|Texas Instruments Incorporated
| 3-Line To 8-Line decoder/Demultiplexer
| Marketing part#   Digital Voltage Range   Package-type   #pins
| SN74LVC138AD   1.65V - 3.6V   SOIC   16
| SN74LVC138ADBR   1.65V - 3.6V   SSOP   16
| SN74LVC138ADBRE4   1.65V - 3.6V   SSOP   16
| SN74LVC138ADBRG4   1.65V - 3.6V   SSOP   16
| SN74LVC138ADE4   1.65V - 3.6V   SOIC   16
| SN74LVC138ADG4   1.65V - 3.6V   SOIC   16
| SN74LVC138ADGVR   1.65V - 3.6V   TVSOP   16
| SN74LVC138ADGVRE4  1.65V - 3.6V   TVSOP   16
| SN74LVC138ADGVRG4  1.65V - 3.6V   TVSOP   16
| SN74LVC138ADR   1.65V - 3.6V   SOIC   16
| SN74LVC138ADRE4   1.65V - 3.6V   SOIC   16
| SN74LVC138ADRG4   1.65V - 3.6V   SOIC   16
| SN74LVC138ADT   1.65V - 3.6V   SOIC   16
| SN74LVC138ADTE4   1.65V - 3.6V   SOIC   16
| SN74LVC138ADTG4   1.65V - 3.6V   SOIC   16
| SN74LVC138AGQNR   1.65V - 3.6V   BGA MICROSTAR JUNIOR  20
| SN74LVC138ANSR   1.65V - 3.6V   SO   16
| SN74LVC138ANSRE4   1.65V - 3.6V   SO   16
| SN74LVC138ANSRG4   1.65V - 3.6V   SO   16
| SN74LVC138APW   1.65V - 3.6V   TSSOP   16
| SN74LVC138APWE4   1.65V - 3.6V   TSSOP   16
| SN74LVC138APWG4   1.65V - 3.6V   TSSOP   16
| SN74LVC138APWR   1.65V - 3.6V   TSSOP   16
| SN74LVC138APWRE4   1.65V - 3.6V   TSSOP   16
| SN74LVC138APWRG4   1.65V - 3.6V   TSSOP   16
| SN74LVC138APWT   1.65V - 3.6V   TSSOP   16
| SN74LVC138APWTE4   1.65V - 3.6V   TSSOP   16
| SN74LVC138APWTG4   1.65V - 3.6V   TSSOP   16
| SN74LVC138ARGYR   1.65V - 3.6V   VQFN   16
| SN74LVC138ARGYRG4  1.65V - 3.6V   VQFN   16
| SN74LVC138AZQNR   1.65V - 3.6V   BGA MICROSTAR JUNIOR  20
[IBIS Ver]   3.2
[File name]   sn74lvc138a.ibs
[File Rev]   1.0
[Date]   6/21/2012
[Source]
| Texas Instruments Incorporated.
| Analog-eLab Design Center, HPA
| 12500 TI Blvd
| Dallas, TX -75243
| e-mail: elab_scm_ibis@list.ti.com
[Notes]   Revision History:
| Rev 1.0: 6/21/2012
| - Initial version of the model
| - Model generated from simulations in TISPICE
| - Model matched to SPICE simulation
| - C_comp although listed in numerical order of value are
|   obtained from varying PVT conditions. For PVT conditions for
|   each specific value refer the buffer description under
|   respective [Model]. IBIS model user is responsible for using
|   appropriate C_comp to simulate for Signal Integrity.
| - Model names with a trailing _1p8 contains the model for
|   1.8V [1.71V and 1.89V]. Model names with a trailing _3p3
|   contains the model for 3.3V [3.0V and 3.6V].
[Disclaimer]
| This model is designed as an aid for customers of Texas Instruments.
| TI and its licensors and suppliers make no warranties, either expressed
| or implied, with respect to this  model, including the warranties of
| merchantability or fitness for a particular purpose. The model is
| provided solely on an "as is" basis. The entire risk as to its quality
| and performance is with the customer.
[Copyright]
(C) Copyright 2012 Texas Instruments Incorporated.All rights reserved.
|   SN74LVC138ARGY
[Component]   SN74LVC138ARGY
[Manufacturer]   TI
[Package]   |16 VQFN   -  RGY package
|   typ   min   max
R_pkg   0.07181   0.06369   0.08091
L_pkg   1.28975nH   1.12199nH   1.48239nH
C_pkg   0.23145pF   0.21992pF   0.24704pF
[Pin]  signal_name   model_name   R_pin   L_pin   C_pin
1   A   INPUT   0.08031   1.46839nH  0.22398pF
2   B   INPUT   0.08091   1.48239nH  0.23668pF
3   C   INPUT   0.07045   1.26496nH  0.23607pF
4   _G2A   INPUT   0.06569   1.16779nH  0.22308pF
5   _G2B   INPUT   0.06369   1.12697nH  0.22065pF
6   G1   INPUT   0.06587   1.17112nH  0.23290pF
7   Y7   OUTPUT   0.07968   1.45609nH  0.24704pF
8   GND   GND   0.08286   1.52103nH  0.24643pF
9   Y6   OUTPUT   0.07976   1.45197nH  0.23427pF
10   Y5   OUTPUT   0.07984   1.45159nH  0.23652pF
11   Y4   OUTPUT   0.06755   1.19686nH  0.23355pF
12   Y3   OUTPUT   0.06389   1.12199nH  0.22012pF
13   Y2   OUTPUT   0.06405   1.12517nH  0.21992pF
14   Y1   OUTPUT   0.06746   1.19483nH  0.23367pF
15   Y0   OUTPUT   0.07624   1.37643nH  0.24190pF
16   VCC   POWER   0.07919   1.44018nH  0.23234pF
|   SN74LVC138AD
[Component]   SN74LVC138AD
[Manufacturer]   TI
[Package]   |16 SOIC   -  D   package
|   typ   min   max
R_pkg   0.10679   0.08959   0.12155
L_pkg   2.86135nH   2.04402nH   4.29838nH
C_pkg   0.80708pF   0.61580pF   1.19610pF
[Pin]  signal_name   model_name   R_pin   L_pin   C_pin
1   A   INPUT   0.10965   4.21181nH  1.19116pF
2   B   INPUT   0.11559   3.48714nH  0.97723pF
3   C   INPUT   0.10942   2.29983nH  0.63814pF
4   _G2A   INPUT   0.09310   2.09121nH  0.61836pF
5   _G2B   INPUT   0.08959   2.04402nH  0.61580pF
6   G1   INPUT   0.10155   2.19279nH  0.63325pF
7   Y7   OUTPUT   0.11898   3.56208nH  0.96757pF
8   GND   GND   0.11687   4.32168nH  1.19555pF
9   Y6   OUTPUT   0.11525   4.29838nH  1.19610pF
10   Y5   OUTPUT   0.12155   3.59908nH  0.97047pF
11   Y4   OUTPUT   0.10999   2.31319nH  0.63900pF
12   Y3   OUTPUT   0.09528   2.12402nH  0.61985pF
13   Y2   OUTPUT   0.09454   2.11191nH  0.61892pF
14   Y1   OUTPUT   0.10669   2.26123nH  0.63716pF
15   Y0   OUTPUT   0.11386   3.46224nH  0.97610pF
16   VCC   POWER   0.10996   4.21621nH  1.19058pF
|   SN74LVC138ANS
[Component]   SN74LVC138ANS
[Manufacturer]   TI
[Package]   |16 SO   -  NS  package
|   typ   min   max
R_pkg   0.08605   0.07325   0.09888
L_pkg   3.34130nH   2.45216nH   4.64452nH
C_pkg   0.44622pF   0.34335pF   0.59414pF
[Pin]  signal_name   model_name   R_pin   L_pin   C_pin
1   A   INPUT   0.09452   4.54808nH  0.58389pF
2   B   INPUT   0.09261   3.98297nH  0.53721pF
3   C   INPUT   0.08490   2.91391nH  0.38240pF
4   _G2A   INPUT   0.07560   2.49736nH  0.34550pF
5   _G2B   INPUT   0.07325   2.45216nH  0.34335pF
6   G1   INPUT   0.07916   2.80448nH  0.37892pF
7   Y7   OUTPUT   0.09443   4.02551nH  0.54091pF
8   GND   GND   0.10023   4.67424nH  0.59337pF
9   Y6   OUTPUT   0.09888   4.64452nH  0.59414pF
10   Y5   OUTPUT   0.09698   4.07805nH  0.54351pF
11   Y4   OUTPUT   0.08555   2.93340nH  0.38459pF
12   Y3   OUTPUT   0.07766   2.54090nH  0.34744pF
13   Y2   OUTPUT   0.07715   2.52880nH  0.34648pF
14   Y1   OUTPUT   0.08314   2.87924nH  0.38239pF
15   Y0   OUTPUT   0.09088   3.94883nH  0.53633pF
16   VCC   POWER   0.09477   4.54868nH  0.58420pF
|   SN74LVC138ADB
[Component]   SN74LVC138ADB
[Manufacturer]   TI
[Package]   |16 SSOP   -  DB  package
|   typ   min   max
R_pkg   0.14054   0.11842   0.16244
L_pkg   3.29871nH   2.75952nH   4.11419nH
C_pkg   0.48137pF   0.45298pF   0.52751pF
[Pin]  signal_name   model_name   R_pin   L_pin   C_pin
1   A   INPUT   0.15054   4.01919nH  0.52150pF
2   B   INPUT   0.15621   3.49194nH  0.49024pF
3   C   INPUT   0.13675   3.19930nH  0.47605pF
4   _G2A   INPUT   0.12151   2.80361nH  0.45481pF
5   _G2B   INPUT   0.11842   2.75952nH  0.45298pF
6   G1   INPUT   0.12992   3.10167nH  0.47342pF
7   Y7   OUTPUT   0.15856   3.53752nH  0.49134pF
8   GND   GND   0.15895   4.14749nH  0.52726pF
9   Y6   OUTPUT   0.15674   4.11419nH  0.52751pF
10   Y5   OUTPUT   0.16244   3.59622nH  0.49427pF
11   Y4   OUTPUT   0.13853   3.23037nH  0.47855pF
12   Y3   OUTPUT   0.12466   2.85202nH  0.45683pF
13   Y2   OUTPUT   0.12399   2.84071nH  0.45589pF
14   Y1   OUTPUT   0.13567   3.18360nH  0.47665pF
15   Y0   OUTPUT   0.15357   3.45204nH  0.48920pF
16   VCC   POWER   0.15101   4.02609nH  0.52108pF
|   SN74LVC138APW
[Component]   SN74LVC138APW
[Manufacturer]   TI
[Package]   |16 TSSOP  -  PW  package
|   typ   min   max
R_pkg   0.21641   0.19307   0.24285
L_pkg   3.23731nH   2.84267nH   3.90329nH
C_pkg   0.46631pF   0.43231pF   0.52656pF
[Pin]  signal_name   model_name   R_pin   L_pin   C_pin
1   A   INPUT   0.20625   3.80511nH  0.52181pF
2   B   INPUT   0.23202   3.42299nH  0.49528pF
3   C   INPUT   0.21967   3.07538nH  0.43503pF
4   _G2A   INPUT   0.19810   2.88474nH  0.43805pF
5   _G2B   INPUT   0.19307   2.84267nH  0.43635pF
6   G1   INPUT   0.20861   2.98284nH  0.43231pF
7   Y7   OUTPUT   0.23642   3.46720nH  0.49672pF
8   GND   GND   0.22089   3.93774nH  0.52662pF
9   Y6   OUTPUT   0.21706   3.90329nH  0.52656pF
10   Y5   OUTPUT   0.24285   3.52003nH  0.50025pF
11   Y4   OUTPUT   0.22319   3.10879nH  0.43727pF
12   Y3   OUTPUT   0.20371   2.93421nH  0.44002pF
13   Y2   OUTPUT   0.20263   2.92399nH  0.43922pF
14   Y1   OUTPUT   0.21858   3.06631nH  0.43549pF
15   Y0   OUTPUT   0.22764   3.38481nH  0.49391pF
16   VCC   POWER   0.20705   3.81262nH  0.52140pF
|   SN74LVC138ADGV
[Component]   SN74LVC138ADGV
[Manufacturer]   TI
[Package]   |16 TVSOP  -  DGV package
|   typ   min   max
R_pkg   0.15470   0.14385   0.16940
L_pkg   2.49816nH   2.28613nH   2.93307nH
C_pkg   0.57112pF   0.55387pF   0.59810pF
[Pin]  signal_name   model_name   R_pin   L_pin   C_pin
1   A   INPUT   0.15874   2.93307nH  0.55479pF
2   B   INPUT   0.16940   2.65840nH  0.59810pF
3   C   INPUT   0.15913   2.41485nH  0.56691pF
4   _G2A   INPUT   0.14914   2.32879nH  0.56231pF
5   _G2B   INPUT   0.14385   2.28613nH  0.56023pF
6   G1   INPUT   0.14729   2.31923nH  0.56303pF
7   Y7   OUTPUT   0.16619   2.63538nH  0.59689pF
8   GND   GND   0.16617   2.99524nH  0.55637pF
9   Y6   OUTPUT   0.15715   2.92064nH  0.55387pF
10   Y5   OUTPUT   0.16662   2.63888nH  0.59717pF
11   Y4   OUTPUT   0.15132   2.35285nH  0.56419pF
12   Y3   OUTPUT   0.14407   2.28825nH  0.55995pF
13   Y2   OUTPUT   0.14446   2.29074nH  0.55993pF
14   Y1   OUTPUT   0.15108   2.34858nH  0.56446pF
15   Y0   OUTPUT   0.15739   2.55840nH  0.59379pF
16   VCC   POWER   0.15558   2.90687nH  0.55311pF
|   SN74LVC138AGQN
[Component]   SN74LVC138AGQN
[Manufacturer]   TI
[Package]   |20 BGA MICROSTAR JUNIOR   -  GQN package
|   typ   min   max
R_pkg   0.07324   0.04966   0.12440
L_pkg   1.01804nH   0.68951nH   1.78735nH
C_pkg   0.21885pF   0.17417pF   0.29832pF
[Pin]  signal_name   model_name   R_pin   L_pin   C_pin
A1   B   INPUT   0.06933   1.04408nH  0.22203pF
A2   A   INPUT   0.09242   1.25703nH  0.20954pF
A3   VCC   POWER   0.09416   1.05389nH  0.20244pF
A4   Y0   OUTPUT   0.06717   1.02769nH  0.17417pF
B1   C   INPUT   0.05432   0.78173nH  0.18991pF
B4   Y1   OUTPUT   0.05389   0.77877nH  0.17686pF
C1   _G2B   INPUT   0.04966   0.68951nH  0.18917pF
C2   _G2A   INPUT   0.09161   1.11902nH  0.25931pF
C3   Y3   OUTPUT   0.09192   1.10591nH  0.25841pF
C4   Y2   OUTPUT   0.05102   0.72970nH  0.18784pF
D1   G1   INPUT   0.05063   0.69860nH  0.19305pF
D4   Y4   OUTPUT   0.05521   0.79986nH  0.19204pF
E1   GND   GND   0.08248   1.28341nH  0.30807pF
E2   Y7   OUTPUT   0.10094   1.33631nH  0.27050pF
E3   Y6   OUTPUT   0.12440   1.78735nH  0.29832pF
E4   Y5   OUTPUT   0.07278   1.09695nH  0.24277pF
|   Model Selectors
[Model Selector] INPUT
input_1p8   1.8V  digital input
input_3p3   3.3V  digital input
[Model Selector] OUTPUT
output_1p8   1.8V  digital output
output_3p3   3.3V  digital output
| Models and submodels in the file (4): input_1p8 (Input), input_3p3 (Input), output_1p8 (Output), output_3p3 (Output)
